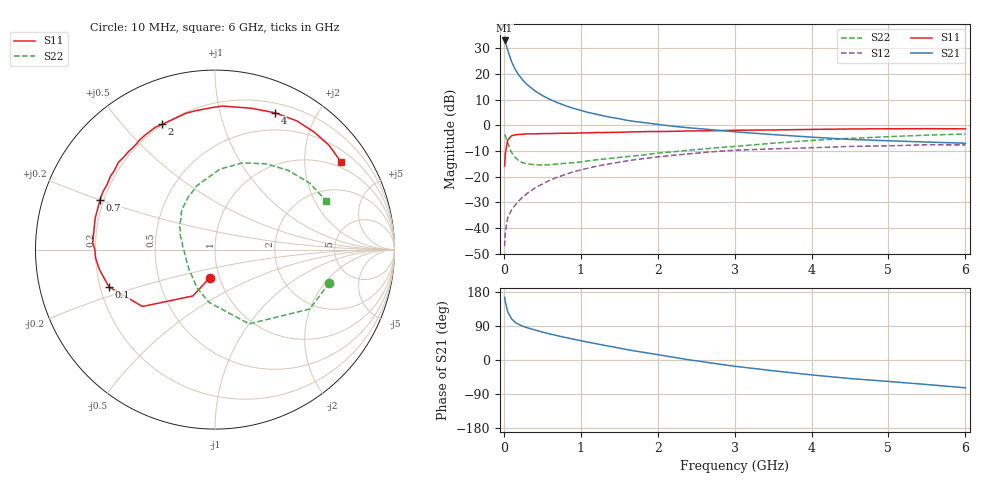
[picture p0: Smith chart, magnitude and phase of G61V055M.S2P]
! SIEMENS Small Signal Semiconductors
! BFG193
! Si NPN RF Bipolar Junction Transistor in SOT223
! VCE = 1 V  IC = 55 mA
! Common Emitter S-Parameters:  August  1996
# GHz  S  MA  R  50
!  f  S11  S21  S12  S22
! GHz  MAG  ANG  MAG  ANG  MAG  ANG  MAG  ANG
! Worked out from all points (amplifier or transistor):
!   36 points, 10 MHz to 6 GHz, reference 50 ohm
!   highest |S21| = 33.1 dB at 10 MHz (marker M1)
!   |S21| within 3 dB of that: start of sweep to 42.32 MHz
!   unconditionally stable (mu >= 1): start of sweep to 15.32 MHz; 188.9 MHz to end of sweep
!   at 250 MHz: K = 1.08, MAG = 21.0 dB, |S12| = -27.9 dB
!   at 1.4 GHz: K = 1.15, MAG = 6.6 dB, |S12| = -14.9 dB
!   at 6 GHz: K = 1.05, MAG = -1.0 dB, |S12| = -7.6 dB
!   S11 on the Smith chart (normalised r, x): 10 MHz: 0.90, -0.29; 100 MHz: 0.24, -0.16; 700 MHz: 0.19, +0.20; 2 GHz: 0.20, +0.65; 4 GHz: 0.30, +1.49; 6 GHz: 0.83, +2.99
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0.01  0.1604 -100.8  45.24 165.6  0.0044 75.4  0.6639 -16.2
0.02  0.2861 -115.5  41.69 153.3  0.0083 68.0  0.6232 -32.1
0.05  0.5136 -141.9  29.25 127.3  0.0158 57.5  0.4554 -65.3
0.1  0.6264 -160.7  17.55 108.8  0.0224 55.8  0.296 -96.3
0.15  0.6532 -170.2  12.17 99.1  0.0283 57.3  0.235 -115.7
0.2  0.6667 -175.9  9.322 93.4  0.0341 61.2  0.2012 -127.4
0.25  0.6701 179.9  7.497 88.9  0.0402 62.7  0.1855 -139.3
0.3  0.6818 176.7  6.297 85.4  0.0467 63.9  0.1778 -146.4
0.4  0.6832 170.7  4.753 79.5  0.0594 64.4  0.1702 -159.4
0.5  0.69 165.5  3.818 73.8  0.0718 63.8  0.1683 -168.7
0.6  0.6918 161.2  3.198 68.8  0.0851 62.8  0.1705 -175.1
0.7  0.6978 156.7  2.76 63.9  0.0977 61.2  0.1763 179.0
0.9  0.7019 148.9  2.159 55.2  0.1235 57.3  0.1864 167.8
1.1  0.7129 141.8  1.781 46.9  0.1467 53.1  0.2034 160.3
1.6  0.7409 124.6  1.254 27.6  0.2028 41.0  0.2458 142.2
2  0.7574 112.9  1.043 14.3  0.242 31.0  0.2882 129.9
2.2  0.7633 107.4  0.961 7.5  0.2608 26.0  0.3037 123.8
3.5  0.8132 75.6  0.66 -28.3  0.3488 -7.1  0.4491 86.5
4  0.8322 66.3  0.589 -39.3  0.3652 -16.8  0.508 72.2
4.5  0.8497 57.6  0.531 -48.9  0.3885 -26.7  0.5568 59.0
5.5  0.8612 42.3  0.472 -64.7  0.4177 -49.0  0.6447 35.1
6  0.8552 34.7  0.448 -73.4  0.4152 -61.6  0.6767 23.6
